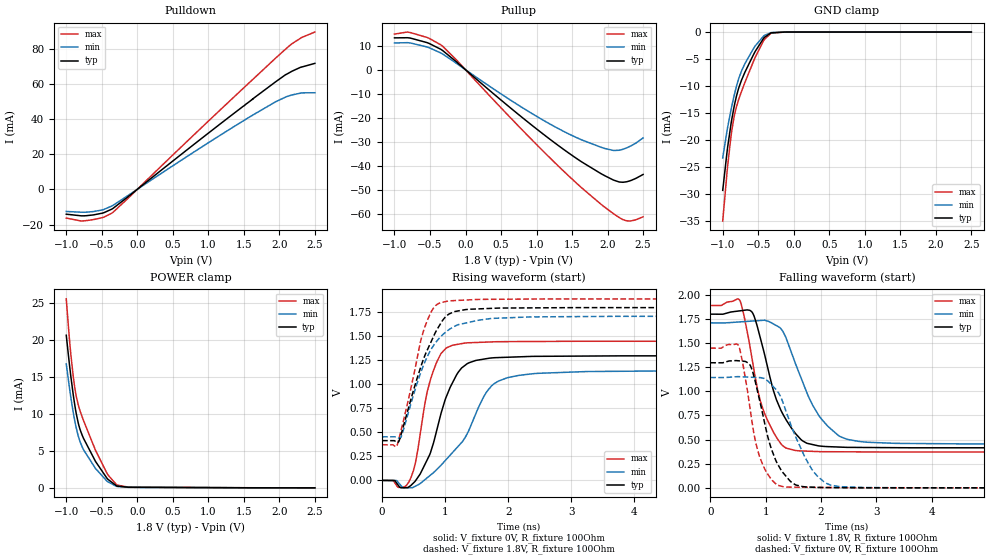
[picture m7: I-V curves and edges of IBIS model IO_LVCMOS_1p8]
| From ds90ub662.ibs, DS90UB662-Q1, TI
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|   IO_LVCMOS_1p8   Model
[Model]   IO_LVCMOS_1p8
Model_type   I/O
Polarity   Non-Inverting
Enable   Active-Low
Vinl = 0.54
Vinh = 1.26
Vmeas = 0.9
Vref = 0
Cref = 1pF
Rref = 100000
|   typ   min   max
C_comp   0.362pF   0.313pF   0.461pF
[Voltage Range]   1.8   1.71   1.89
[Temperature Range]   27   105   -40
[Pullup Reference]   1.8   1.71   1.89
[Pulldown Reference]   0   0   0
[Power Clamp Reference]   1.8   1.71   1.89
[GND Clamp Reference]   0   0   0
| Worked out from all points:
|   slope of the pulldown table from 0 to 0.27 V, typ, clamps not added: 31 ohm
|   slope of the pullup table from 0 to 0.27 V, typ, clamps not added: 39.2 ohm
|   GND clamp passes 1 mA (typ) near -0.41 V on its own axis
|   POWER clamp passes 1 mA (typ) near -0.39 V on its own axis
|   falling waveform, V_fixture 1.8V, R_fixture 100Ohm: 20-80 % time 467ps typ, 592ps min, 378ps max; typ from 1.8 V to 0.414 V
|   rising waveform, V_fixture 0V, R_fixture 100Ohm: 20-80 % time 384ps typ, 620ps min, 265ps max; typ from 0 V to 1.3 V
|   rising waveform, V_fixture 1.8V, R_fixture 100Ohm: 20-80 % time 440ps typ, 462ps min, 314ps max; typ from 0.414 V to 1.8 V
|   falling waveform, V_fixture 0V, R_fixture 100Ohm: 20-80 % time 366ps typ, 505ps min, 287ps max; typ from 1.3 V to 0 V
[Pulldown]
|   Voltage   I(typ)   I(min)   I(max)
-1V       -14.12mA   -12.57mA   -16.32mA
-790mV    -15.05mA   -13mA      -18mA
-723.5mV  -15mA      -12.99mA   -17.8mA
-492.5mV  -13.54mA   -11.69mA   -16.08mA
-345.5mV  -10.91mA   -9.183mA   -13.15mA
1.051V    33.53mA    27.78mA    40.7mA
1.541V    48.74mA    40.13mA    59.28mA
1.947V    61.11mA    49.77mA    74.57mA
2.091V    65.25mA    52.5mA     79.81mA
2.171V    66.98mA    53.6mA     82.58mA
2.321V    69.61mA    54.85mA    86.45mA
2.5V      71.6mA     54.91mA    89.43mA
[GND Clamp]
|   Voltage   I(typ)   I(min)   I(max)
-1V       -29.31mA   -23.3mA    -34.99mA
-937mV    -21.95mA   -18.1mA    -25.64mA
-884.5mV  -17.12mA   -14.49mA   -19.42mA
-839mV    -13.77mA   -11.75mA   -15.64mA
-807.5mV  -11.91mA   -10.09mA   -13.87mA
-772.5mV  -10.28mA   -8.54mA    -12.37mA
-730.5mV  -8.762mA   -7.068mA   -10.82mA
-566mV    -4.16mA    -3.045mA   -5.397mA
-422.5mV  -1.127mA   -714.9uA   -1.563mA
-321mV    -171.5uA   -110.9uA   -237.1uA
-125mV    -5.452uA   -4.994uA   -6.25uA
2.5V      0A         0A         0A
[Pullup]
|   Voltage   I(typ)   I(min)   I(max)
-1V       13.2mA     11.08mA    14.77mA
-779.5mV  13.13mA    11.1mA     15.43mA
-513.5mV  10.9mA     9.112mA    13.03mA
-321mV    7.9mA      6.45mA     9.695mA
858.5mV   -21.4mA    -16.93mA   -26.98mA
1.275V    -30.95mA   -24.08mA   -39.28mA
1.635V    -38.46mA   -29.28mA   -49.26mA
1.961V    -44.21mA   -32.86mA   -57.34mA
2.08V     -45.97mA   -33.68mA   -59.95mA
2.16V     -46.79mA   -33.61mA   -61.57mA
2.3V      -46.48mA   -32.19mA   -63.08mA
2.5V      -43.69mA   -28.48mA   -61.33mA
[POWER Clamp]
|   Voltage   I(typ)   I(min)   I(max)
-1V       20.61mA    16.74mA    25.52mA
-954.5mV  16.6mA     13.48mA    19.96mA
-933.5mV  14.91mA    12.1mA     17.83mA
-902mV    12.61mA    10.21mA    15.09mA
-870.5mV  10.63mA    8.586mA    12.96mA
-832mV    8.785mA    7.035mA    11.23mA
-755mV    6.647mA    5.12mA     9.047mA
-587mV    3.552mA    2.602mA    5.05mA
-429.5mV  1.332mA    936uA      2.012mA
-293mV    275.2uA    206.9uA    433.3uA
-125mV    79.86uA    66.69uA    99.13uA
2.5V      0A         0A         0A
[Ramp]
R_load = 100
|   typ   min   max
dV/dt_r   0.778029/3.80291e-10   0.686721/6.21269e-10   0.868834/2.63781e-10
dV/dt_f   0.831489/4.65612e-10   0.753509/5.91452e-10   0.91145/3.76613e-10
[Falling Waveform]
V_fixture = 1.8V
V_fixture_min = 1.71V
V_fixture_max = 1.89V
R_fixture = 100Ohm
C_fixture = 0F
|   Time   V(typ)   V(min)   V(max)
0s        1.8V       1.71V      1.89V
531.9ps   1.834V     1.72V      1.944V
753.8ps   1.821V     1.728V     1.341V
903.6ps   1.554V     1.734V     902.4mV
1.063ns   1.183V     1.723V     665.5mV
1.314ns   761.5mV    1.619V     434.5mV
1.53ns    570.4mV    1.302V     387.9mV
2.122ns   427.2mV    639.4mV    374.5mV
2.853ns   418.1mV    472.2mV    372.4mV
20ns      414.1mV    454.1mV    370.8mV
[Rising Waveform]
V_fixture = 0V
V_fixture_min = 0V
V_fixture_max = 0V
R_fixture = 100Ohm
C_fixture = 0F
|   Time   V(typ)   V(min)   V(max)
0s        4.537uV    10.01uV    2.362uV
354.7ps   -75.88mV   -77.29mV   -67.73mV
527.8ps   -6.194mV   -60.18mV   180.8mV
704.4ps   199.5mV    21.03mV    887.2mV
861.2ps   506.6mV    109.7mV    1.222V
1.081ns   970.3mV    263.7mV    1.397V
1.304ns   1.192V     433.9mV    1.429V
1.736ns   1.275V     984.5mV    1.442V
2.476ns   1.292V     1.115V     1.446V
20ns      1.297V     1.145V     1.448V
[Rising Waveform]
V_fixture = 1.8V
V_fixture_min = 1.71V
V_fixture_max = 1.89V
R_fixture = 100Ohm
C_fixture = 0F
|   Time   V(typ)   V(min)   V(max)
0s        414.1mV    454.1mV    370.9mV
237.8ps   395.4mV    449.1mV    363.4mV
306.3ps   488.9mV    458.7mV    536mV
608.3ps   1.17V      1.112V     1.439V
675.3ps   1.294V     1.227V     1.592V
840ps     1.533V     1.427V     1.814V
1.047ns   1.726V     1.563V     1.867V
1.522ns   1.785V     1.667V     1.884V
2.351ns   1.796V     1.702V     1.888V
20ns      1.8V       1.71V      1.89V
[Falling Waveform]
|Gnd
V_fixture = 0V
V_fixture_min = 0V
V_fixture_max = 0V
R_fixture = 100Ohm
C_fixture = 0F
|   Time   V(typ)   V(min)   V(max)
0s        1.296V     1.143V     1.448V
511.6ps   1.317V     1.152V     1.475V
719.4ps   1.271V     1.147V     818.4mV
825.4ps   1.07V      1.144V     457mV
943.9ps   773.6mV    1.138V     244.9mV
1.102ns   405.5mV    1.071V     89.67mV
1.331ns   145.8mV    855.4mV    9.757mV
1.827ns   7.147mV    199mV      5.245mV
2.351ns   2.154mV    13.02mV    2.28mV
20ns      4.85uV     11uV       2.393uV
